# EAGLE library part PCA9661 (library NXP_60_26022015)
The PCA9661 is an advanced single master mode I2C-bus controller. It is a fourth generation bus controller designed for data intensive I2C-bus data transfers. AAL Eindhoven MK
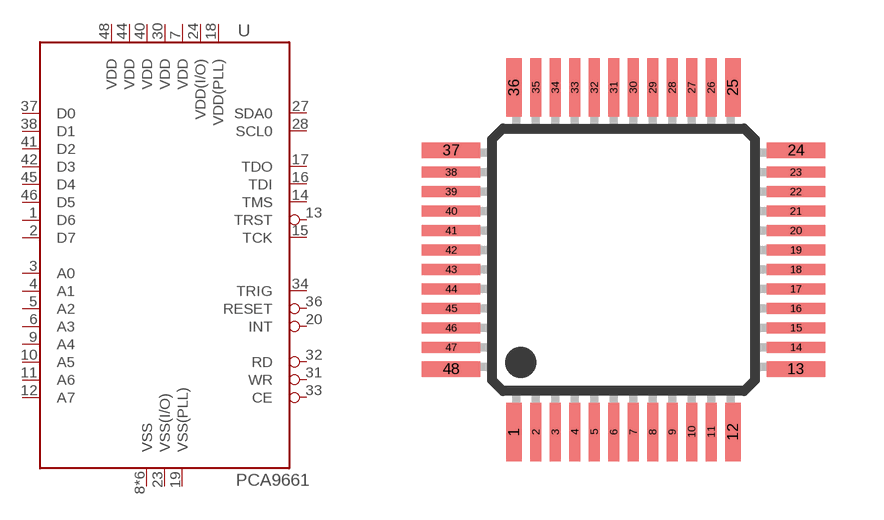
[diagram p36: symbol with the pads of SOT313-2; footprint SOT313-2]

Designator prefix U

## PCA9661B  [SOT313-2]
1  D6
2  D7
3  A0  in
4  A1  in
5  A2  in
6  A3  in
7  VDD  pwr
8  VSS  pwr
9  A4  in
10  A5  in
11  A6  in
12  A7  in
13  TRST  in
14  TMS  in
15  TCK  in
16  TDI  in
17  TDO  out
18  VDD(PLL)  pwr
19  VSS(PLL)  pwr
20  INT  out
23  VSS(I/O)  pwr
24  VDD(I/O)  pwr
27  SDA0
28  SCL0
29  VSS  pwr
30  VDD  pwr
31  WR  in
32  RD  in
33  CE  in
34  TRIG  in
35  VSS  pwr
36  RESET  in
37  D0
38  D1
39  VSS  pwr
40  VDD  pwr
41  D2
42  D3
43  VSS  pwr
44  VDD  pwr
45  D4
46  D5
47  VSS  pwr
48  VDD  pwr

## Footprint SOT313-2 (pad centres in mm)
SOT313-2 LQFP48: plastic low profile quad flat package; 48 leads; body 7 x 7 x 1.4 mm JEDEC: MS-026 IEC: 136E05 Footprint according to NXP SOT313-2 specification, however the cornerpins are 0.4mm in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
smd 0.4 x 1.5: 1 -2.81,-4.425; 12 2.81,-4.425; 25 2.81,4.425; 36 -2.81,4.425
smd 0.28 x 1.5: 2 -2.25,-4.425; 3 -1.75,-4.425; 4 -1.25,-4.425; 5 -0.75,-4.425; 6 -0.25,-4.425; 7 0.25,-4.425; 8 0.75,-4.425; 9 1.25,-4.425; 10 1.75,-4.425; 11 2.25,-4.425; 26 2.25,4.425; 27 1.75,4.425; 28 1.25,4.425; 29 0.75,4.425; 30 0.25,4.425; 31 -0.25,4.425; 32 -0.75,4.425; 33 -1.25,4.425; 34 -1.75,4.425; 35 -2.25,4.425
smd 1.5 x 0.4: 13 4.425,-2.81; 24 4.425,2.81; 37 -4.425,2.81; 48 -4.425,-2.81
smd 1.5 x 0.28: 14 4.425,-2.25; 15 4.425,-1.75; 16 4.425,-1.25; 17 4.425,-0.75; 18 4.425,-0.25; 19 4.425,0.25; 20 4.425,0.75; 21 4.425,1.25; 22 4.425,1.75; 23 4.425,2.25; 38 -4.425,2.25; 39 -4.425,1.75; 40 -4.425,1.25; 41 -4.425,0.75; 42 -4.425,0.25; 43 -4.425,-0.25; 44 -4.425,-0.75; 45 -4.425,-1.25; 46 -4.425,-1.75; 47 -4.425,-2.25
